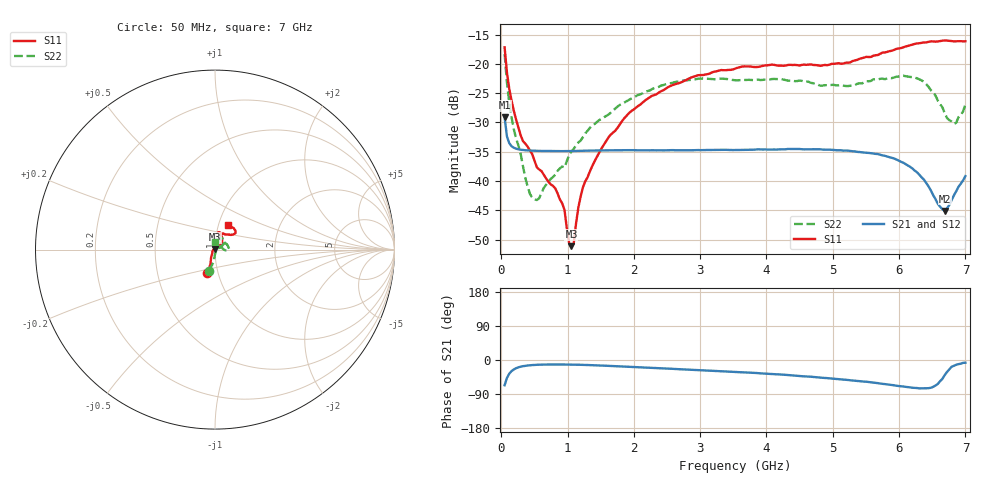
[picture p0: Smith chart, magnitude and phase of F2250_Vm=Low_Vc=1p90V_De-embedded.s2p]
! Integrated Device Technology
! Corporate Headquarters
! 6024 Silver Creek Valley Road
! San Jose, CA 95138  USA
! Phone:  1-408-284-8200
! Toll Free:  1-800-223-1366
! Webpage:  http://www.idt.com/
! Timing and RF Division
! 515 Groton Road, Suite 102
! Westford, MA 01886-6024
! Device:  F2250
! Description: Voltage Variable RF Attenuator
! Frequency:  50.0 -  6000.00 MHz
! Package:  3x3 mm Thin QFN Plastic Package: 16 pin
! Ports:  2 RF, 3 DC
!  Pin  1  = GND
!  Pin  2  = NC
!  Pin  3  = RF1  = Port 1
!  Pin  4  = NC
!  Pin  5  = GND
!  Pin  6  = GND
!  Pin  7  = GND
!  Pin  8  = GND
!  Pin  9  = NC
!  Pin 10  = RF2  = Port 2
!  Pin 11  = NC
!  Pin 12  = GND
!  Pin 13  = GND
!  Pin 14  = VCNTRL
!  Pin 15  = VDD
!  Pin 16  = VMODE
! Vcntrl:  1.900 Volts
! Vmode:  +0.000 Volts
! Vdd:  +3.30  Volts
! Current:  1.182 mA
! Data:  The device was measured on a the F2250 evaluation board which has
!  individual transmission lines to the RF pins.  Data was collected
!  using a calibrated network analyzer.  The evaluation board was
!  de-embedded using a TRL calibration technique.
!  The reference plane is the edge of the package pin.
! Misc:  SN 10
!  Action Tracker AT0258
! Date Measured:  2014-11-26
! Date:  2015-10-15  MJV
! Note:
!  Integrated Device Technology supplies this data as a sample of measured
!  data at the package pin for this product.  Your particular data for this
!  product may vary.
!  Data was taken at 25 degrees C.
!  Integrated Device Technology reserves the right to change this data at anytime.
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# GHz S dB R 50
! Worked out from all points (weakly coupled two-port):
!   201 points, 50 MHz to 7 GHz, reference 50 ohm
!   highest |S21| = -29.11 dB at 50 MHz (marker M1); lowest = -45.1 dB at 6.687 GHz (marker M2)
!   lowest |S11| = -51.1 dB at 1.058 GHz (marker M3), VSWR 1.01, Z = 49.9 + j0.24 ohm
!   |S11| at or under -10 dB: start of sweep to end of sweep
!   |S22| runs from -43.2 to -18.3 dB; largest |S21 - S12| = 5.5e-05
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0.05  -17.17 -108.5  -29.11 -66.6  -29.11 -66.6  -18.31 -105.5
0.08475  -21.44 -107.3  -32.36 -47.6  -32.37 -47.5  -23.11 -96.5
0.189  -28.01 -119.4  -34.31 -24.8  -34.31 -24.8  -31.16 -90.5
0.328  -33.20 -133.3  -34.70 -16.3  -34.70 -16.3  -37.52 -67.3
0.467  -35.43 -146.9  -34.81 -13.4  -34.81 -13.3  -42.85 -30.5
0.57125  -38.02 -160.0  -34.85 -12.4  -34.85 -12.4  -42.92 -8.7
0.91875  -43.80 158.1  -34.89 -11.9  -34.89 -11.9  -37.51 17.9
0.9535  -44.92 169.7  -34.89 -11.9  -34.89 -11.9  -37.68 24.0
1.023  -50.57 143.6  -34.88 -12.1  -34.88 -12.1  -35.54 24.7
1.05775  -51.11 120.3  -34.88 -12.1  -34.88 -12.1  -34.95 26.0
1.0925  -50.63 87.5  -34.87 -12.2  -34.87 -12.2  -34.50 25.0
1.162  -44.55 55.1  -34.85 -12.5  -34.84 -12.5  -33.42 22.3
1.2315  -41.07 43.1  -34.83 -12.8  -34.83 -12.8  -32.49 21.0
1.6485  -32.09 41.6  -34.77 -15.6  -34.76 -15.6  -28.35 29.2
2.37825  -24.88 47.2  -34.74 -21.6  -34.74 -21.7  -23.89 36.8
3.525  -20.82 72.4  -34.70 -31.5  -34.70 -31.5  -22.78 62.9
4.7065  -20.18 72.3  -34.56 -44.8  -34.56 -44.8  -23.31 65.2
5.85325  -17.82 40.4  -35.92 -65.1  -35.91 -65.2  -22.41 11.3
6.33975  -16.41 40.9  -39.37 -74.8  -39.38 -74.9  -22.81 -2.8
6.68725  -15.99 48.8  -45.11 -40.1  -45.12 -39.7  -28.38 17.1
6.82625  -16.14 53.5  -42.45 -15.2  -42.40 -15.1  -30.24 51.7
7  -16.13 63.2  -39.15 -7.2  -39.11 -7.3  -26.91 92.4
